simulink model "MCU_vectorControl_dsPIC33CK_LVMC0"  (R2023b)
settings: Solver=FixedStepDiscrete  StartTime=0.0  StopTime=10.0  FixedStep=5e-5  RelTol=1e-3  EnableMultiTasking=on
undefined symbols (not defined in the file or in its folder): A0, A4, ADC, address, also, AN0, AN1, as, B0, B2, below, Bias1, Bias2, bit, bits, BOR, C12, C13, C14, C7, C8, cause, Code, Communicate, control, counter, Custom, D11, D12, D13, D14, D2, D5, D6, D7, D9, dead, default, deviced, diff, disasserted, DiscIntNeverNeededParam, ECIO, ensure, events, faster, HS3, I, I2C, I2C1, I2C2, I2C3, illegalInstruction, Interval, inverter, is, IsSigned1, IsSigned2, kHz, Lowest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
libraries: simulink x55, MCHP_Blockset x25
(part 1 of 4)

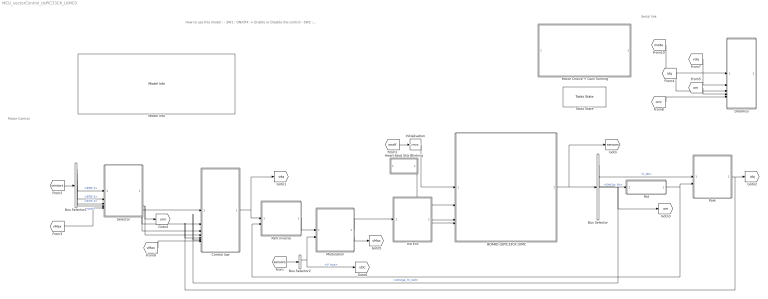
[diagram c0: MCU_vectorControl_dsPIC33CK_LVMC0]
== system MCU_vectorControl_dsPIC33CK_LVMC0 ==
  note: How to use this model : - SW1 : ON/OFF -> Enable or Disable the control - SW2 : mode -> - mode = 0 : Open loop, pot apply a reference voltage in the interval $[0 - V_{\rm max}]$ - mode = 1 : Speed Control, pot apply a reference speed in the intervel $[0 - \Omega_{\rm max}]$ - SW3 : dir : pressing the switch reverse the direction The motor and the control gains can be modified using the block Motor Choice + Gain Tunning
  note: Motor Control
  note: Serial link
  BOARD dsPIC33CK LVMC : Subsystem  mask(dsPIC33CK Low Voltage Motor Control Board (LVMC) - dsPIC33CK256MP508){boardVariants=internal Op-Amp, n=model.p, QEIResolution=4*model.enclines, QEI_Reset=on logical input (software), QEI_Offset_settings=0, QEIOffset=0}
      mask prompts: boardVariants "board variants"; n "Motor poles pairs"; QEIResolution "Optical encoder resolution per mechanical rotation (lines)"; QEI_Reset "Optical encoder reset"; QEI_Offset_settings "Optical encoder offset (mechanical in rad)"; QEIOffset "Optical encoder offset (mechanical in rad)"
      mask help: Template for motor control algorithm. Open subsystem (ctrl-u) for further customisation. Block bus output provices: - Current phase ia & ib, DC bus and potentiometer position - Buttons (0 when pressed) - QEI position and velocity - MCU load and overload Block inputs: - INIT signal average the current phase ia and ib to be removed - LEDs - Reset encoder allows to align the motor while reseting the encoder - PWM normalized duty cycle value Model 50us base rate (20kHz) is synchronized with ADC conversion which is synchronized with the 50us PWM periods
      mask init:
      | BlksQEI = find_system(gcb,'FollowLinks','on','LookUnderMasks','all','ReferenceBlock','MCHP_Blockset/QEI/QEI');
      | QEI_Reset = get_param(gcb,'QEI_Reset');
      | if numel(BlksQEI) >= 1
      |     switch QEI_Reset
      |         case 'on index signal'
      |             set_param(BlksQEI{1},'PIMOD_mode','RESET position on each INDEX event');
      |         case 'on logical input (software)'        
      |             set_param(BlksQEI{1},'PIMOD_mode','position is cyclique between user defined boundaries'); 
      |         case 'custom setting'
      |             % do nothing 
      |     end
      | end % if
      | 
      | 
      |     BlksOpAmp = find_system(gcb,'FollowLinks','on','IncludeCommented','on','LookUnderMasks','all','ReferenceBlock','MCHP_Blockset/Analog IO/Op-Amp');
      |     if numel(BlksOpAmp) >= 1
      |         boardVariants = get_param(gcb,'boardVariants');
      |         switch boardVariants
      |             case 'internal Op-Amp'
      |                 set_param(BlksOpAmp{1},'Commented','off');
      |             case 'external Op-Amp'
      |                 set_param(BlksOpAmp{1},'Commented','on');
      |         end
      |     end % if
  Bus Selector : BusSelector  OutputSignals=ADC.I_ab,optical coder.elec.SinCos_th,optical coder.mecc.omega_m_rad
  Bus Selector1 : BusSelector  OutputSignals=BTN.BTN 1,BTN.BTN 2,BTN.BTN 3,ADC.pot
  Bus Selector2 : BusSelector  OutputSignals=ADC.V_bus
  Control law : Subsystem
  DataVisu : Subsystem
  Heart-beat 5Hz Blinking : Subsystem
  Init Enc : Subsystem
  Initialisation : simulink/Logic and Bit Operations/Compare To Constant  relop===  const=0  OutDataTypeStr=boolean
  Model Info : simulink/Model-Wide Utilities/Model Info  Frame=on  DisplayStringWithTags=|  HorizontalTextAlignment=Center  LeftAlignmentValue=0.5
      | %<ModelName> v%<ModelVersion> - %<Creator>
      | 
      | %<Description>
      | 
      | Last modified on: %<LastModificationDate>
  Modulation : Subsystem  mask{modulation=Space Vector, mod=0}
      mask init:
      | switch modulation
      |     case 'Sinusoidale'
      |         mod = 0;
      |     otherwise
      |         mod = 1;
      | end
  Motor Choice + Gain Tunning : Subsystem  mask(INSA motor control gain tunning){presetMotor=Custom, modelPMSM=Custom, p=5, R=0.2, L=0.00015, Phif=0.0066, J=6e-06, F=1e-05, C0=0, vMax=36, iMax=12, omegaMax=60, enclines=2500, zetaE=0.7, trE=3*model.L/model.R, trWnE=3, KpE=0.08, KiE=-266.6667, zetaM=1.0, trM=3*model.J/model.F/10, trWnM=5, KpM=0.006532, KiM=-0.093528, tsMeca=1e-3}
      mask prompts: presetMotor "Predefined motor"; modelPMSM "PMSM model"; p "Poles pairs p"; R "Phase resistor R (Ohm)"; L "Phase inductance L (H)"; Phif "Flux constant Phif (Wb)"; J "Intertia J (kg.m^2)"; F "Damping coefficient F (N.m.s/rad)"; C0 "Coulomb friction C0 (N.m)"; vMax "Max Voltage (V)"; iMax "Max Current iMax (A)"; omegaMax "Max Speed (rad/s)"; enclines "Lines (RAW)"; zetaE "Damping factor (zeta)"; trE "Time response (s)"; trWnE "TrWn (3 for zeta = 0.7)"; KpE "Kp"; KiE "Ki"; zetaM "Damping factor (zeta)"; trM "Time response (s)"; trWnM "TrWn (3 for zeta = 0.7)"; KpM "Kp"; KiM "Ki"; tsMeca "Mecanical Sampling Time (s)"
      mask help: The bloc provides basic gain tunning solution based on pole placement.
      mask init:
      | % Mototor definition
      | model = struct;
      |          
      | switch presetMotor
      |     case 'Teknic-2310P'
      |         model.modelPMSM    = 'Teknic-2310P';                                 %           // Manufacturer Model Number
      |         model.p        = 4;                                                  %           // Pole Pairs for the motor
      |         model.R        = 0.656;                                              %Ohm        // Stator Resistor
      |         model.L        = 0.35e-3;                                            %H          // Inductance value
      |         model.Phif     = 6.6e-3;                                             %Wb         // PM flux
      |         model.J        = 1e-05;                                              %Kg-m2      // Inertia in SI units
      |         model.F        = 1.e-05;                                             %Kg-m2/s    // Friction Co-efficient
      |         model.C0       = 0.01;                                               %Kg-m2      // Dry friction
      |         model.vMax     = 48;                                                 %V          // Max voltage      
      |         model.iMax     = 10;                                                 %A          // Max current
      |         model.omegaMax = 500;                                                %rad/spm    // Max speed
      |         model.enclines = 1000;                                               % top       // Encoder top per round
      |     case 'Short HURST (AC300020)'
      |         model.modelPMSM    = 'Short HURST (AC300020)';                       %           // Manufacturer Model Number
      |         model.p        = 5;                                                  %           // Pole Pairs for the motor
      |         model.R        = 2.015;                                              %Ohm        // Stator Resistor
      |         model.L        = 2.3e-3;                                             %H          // Inductance value
      |         model.Phif     = 3.3e-3;                                             %Wb         // PM flux
      |         model.J        = 1.908e-04;                                          %Kg-m2      // Inertia in SI units
      |         model.F        = 1.044e-04;                                          %Kg-m2/s    // Friction Co-efficient
      |         model.C0       = 0.01;                                               %Kg-m2      // Dry friction
      |         model.vMax     = 48;                                                 %V          // Max voltage      
      |         model.iMax     = 10;                                                 %A          // Max current
      |         model.omegaMax = 350;                                                %rad/spm    // Max speed    
      |         model.enclines = NaN;                                                % top       // Encoder top per round
      |     case 'Long HURST (AC300022)'
      |         model.modelPMSM    = 'Long HURST (AC300022)';                        %           // Manufacturer Model Number
      |         model.p        = 5;                                                  %           // Pole Pairs for the motor
      |         model.R        = 0.405;                                              %Ohm        // Stator Resistor
      |         model.L        = 0.30e-3;                                            %H          // Inductance value
      |         model.Phif     = 7.63e-3;                                            %Wb         // PM flux
      |         model.J        = 1.908e-04;                                          %Kg-m2      // Inertia in SI units
      |         model.F        = 1.044e-04;                                          %Kg-m2/s    // Friction Co-efficient
      |         model.C0       = 0.01;                                               %Kg-m2      // Dry friction
      |         model.vMax     = 48;                                                 %V          // Max voltage      
      |         model.iMax     = 10;                                                 %A          // Max current
      |         model.omegaMax = 350;                                                %rad/spm    // Max speed    
      |         model.enclines = 250;                                                % top       // Encoder top per round
      |     case 'Custom'
      |         model.modelPMSM    = 'Custom';                                       %           // Manufacturer Model Number
      |         model.p        = p;                                                  %           // Pole Pairs for the motor
      |         model.R        = R;                                                  %Ohm        // Stator Resistor
      |         model.L        = L;                                                  %H          // Inductance value
      |         model.Phif     = Phif;                                               %Wb         // PM flux
      |         model.J        = J;                                                  %Kg-m2      // Inertia in SI units
      |         model.F        = F;                                                  %Kg-m2/s    // Friction Co-efficient
      |         model.C0       = C0;                                                 %Kg-m2      // Dry friction
      |         model.vMax     = vMax;                                               %V          // Max voltage      
      |         model.iMax     = iMax;                                               %A          // Max current
      |         model.omegaMax = omegaMax;                                           %rad/spm    // Max speed
      |         model.enclines = enclines;                                           % top       // Encoder top per round
      | end
      | 
      | 
      | 
      | ff = fields(model);
      | for i=1:numel(ff)
      |     set_param(gcb,ff{i},num2str(model.(ff{i})) );
      | end
      | %% Define fracation length for fixed point datatype
      | model.FracLen.curr  = (15-ceil(log2(model.iMax)));  % Fraction length for current variables
      | model.FracLen.volt  = (15-ceil(log2(model.vMax)));    % Fraction length for voltage variables
      | model.FracLen.volt2 = (15-ceil(log2(2*model.vMax^2))); % Fraction length for voltage square variables
      | model.FracLen.invsqrtvolt = (15-ceil(log2(1/sqrt(model.vMax/4)^2))); % Fraction length for voltage square variables
      | 
      | 
      | %% LUT 1/sqrt(||v_dq||)
      | func = '1./sqrt(x)';
      | xmin = (model.vMax/4)^2; xmax = 2*model.vMax^2;
      | 
      | xdt = sfix(16); xscale = 2^-(15-ceil(log2(xmax)));
      | ydt = sfix(16); yscale = 2^-(15-ceil(log2(1./sqrt(xmin))));
      | rndmeth = 'Floor';
      | errmax = [];
      | nptsmax = [128];
      | spacing = 'even';
      | 
      | %Compute LUT
      | [model.math.LUTintsqrtx,model.math.LUTintsqrty] = fixpt_look1_func_approx(func,xmin,xmax,xdt,xscale,ydt,yscale,rndmeth,errmax,nptsmax,spacing);
      | 
      | 
      | assignin('base','model',model);
      | 
      | %% Define control structure 
      | control = struct;
      | control.tauElec = model.L/model.R;
      | control.kElec = 1/model.R;
      | control.tauMeca = model.J/model.F;
      | control.kMeca = 3/2*model.p*model.Phif/model.F;
      | 
      | 
      | control.trDElec = trE;
      | control.zetaDElec = zetaE;
      | control.trwnDElec = trWnE;
      | control.wnDElec = control.trwnDElec/control.trDElec;
      | control.kE = [(2*control.zetaDElec*control.wnDElec*control.tauElec-1)/control.kElec, ...
      |                 -control.tauElec*control.wnDElec^2/control.kElec];
      | set_param(gcb, 'KpE', num2str(control.kE(1)));
      | set_param(gcb, 'KiE', num2str(control.kE(2)));
      | 
      | control.trDMeca = trM;
      | control.zetaDMeca = zetaM;
      | control.trwnDMeca = trWnM;
      | control.wnDMeca = control.trwnDMeca/control.trDMeca;
      | control.kM = [(2*control.zetaDMeca*control.wnDMeca*control.tauMeca-1)/control.kMeca, ...
      |                 -control.tauMeca*control.wnDMeca^2/control.kMeca];
      | set_param(gcb, 'KpM', num2str(control.kM(1)));
      | set_param(gcb, 'KiM', num2str(control.kM(2)));
      | 
      | control.tsMeca = tsMeca;
      | 
      | assignin('base','control',control);
  Park : Subsystem
  Park inverse : Subsystem
  Rot : Subsystem
  Selector : Subsystem
  Tasks State : MCHP_Blockset/Profiling/Tasks State  TasksPin=E0 D2 D9 C8  MCHP_PORT={Task D1 Running}{Task D1}15:1:E0;{Task D2 Running}{Task D2}15:1:D2;{Task D3 Running}{Task D3}15:1:D9;{Task D4 Running}{Task D4}15:1:C8;  MCHP_MASTERLINK=MCU_vectorControl_dsPIC33CK_LVMC0/BOARD dsPIC33CK LVMC/Microchip Master
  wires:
  Rot/1("cos sin -sin cos ") -> Park/2(P(pth)), Park inverse/2(P(pth))
  Init Enc/1(reset encoder) -> BOARD dsPIC33CK LVMC/4(reset encoder)
  Init Enc/2(PWM [0 1]) -> BOARD dsPIC33CK LVMC/5(PWM [0 1])
  Park inverse/1(xabc) -> Modulation/1("vabc (en V) ")
  Park/1(idq) -> Control law/5(idq), [idq]
  [vMax] -> Selector/5(vMax)
  Modulation/2(vMax) -> [vMax]
  [vMax] -> Control law/7(vMax)
  Selector/1(onoff) -> Control law/1(on/off)
  [omr] -> DataVisu/5(omr)
  [om] -> DataVisu/4(om)
  Selector/4(omr) -> Control law/4(omr), [omr]
  Bus Selector/3 -> Control law/6(om), [om]  "<omega_m_rad>"
  [mode] -> DataVisu/1(mode)
  [idq] -> DataVisu/3(idq)
  [vdq] -> DataVisu/2(vdq)
  Bus Selector2/1 -> Modulation/2(Vdc), [vDC]  "<V_bus>"
  [sensors] -> Bus Selector2/1
  Selector/2(mode) -> Control law/2(mode)
  Selector/3(vdqr) -> Control law/3(vdqr)
  [sensors] -> Bus Selector1/1
  Control law/1(vdq) -> Park inverse/1(xdq), [vdq]
  Bus Selector/2 -> Rot/1(sin cos)  "<SinCos_th>"
  Bus Selector/1 -> Park/1(xab(c))  "<I_ab>"
  BOARD dsPIC33CK LVMC/1(sensors) -> [sensors], Bus Selector/1
  Heart-beat 5Hz Blinking/1(LED1) -> BOARD dsPIC33CK LVMC/2(LED 1)
  [onoff] -> Initialisation/1
  Initialisation/1 -> BOARD dsPIC33CK LVMC/1(INIT)
  Modulation/1(rho_abc [0 1]) -> Init Enc/1(rho_cont)
  Bus Selector1/1 -> Selector/1(toggle on/off)  "<BTN 1>"
  Bus Selector1/2 -> Selector/2(toggle state)  "<BTN 2>"
  Bus Selector1/3 -> Selector/3(toggle dir)  "<BTN 3>"
  Bus Selector1/4 -> Selector/4(pot)  "<pot>"
